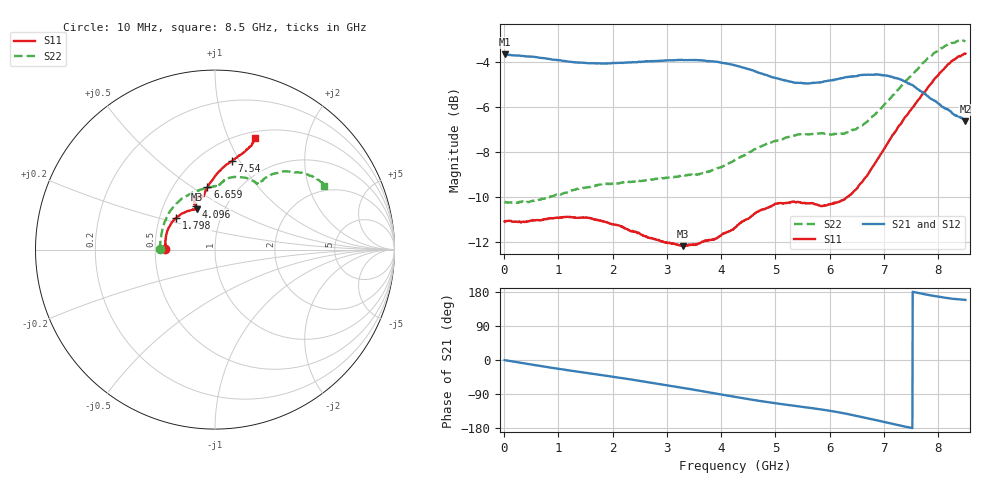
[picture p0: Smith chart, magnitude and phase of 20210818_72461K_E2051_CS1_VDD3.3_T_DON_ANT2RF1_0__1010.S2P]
!Agilent Technologies,E5071C,MY46417908,A.11.23
!Date: Wed Aug 18 14:23:28 2021
!Data & Calibration Information:
!Freq	S11:SOLT2(ON)	S21:SOLT2(ON)	S12:SOLT2(ON)	S22:SOLT2(ON)
!PortZ  Port1:50+j0  Port2:50+j0
!Above PortZ is port z conversion or system Z0 setting when saving the data.
!When reading, reference impedance value at option line is always used.
# Hz S dB R 50
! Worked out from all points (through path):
!   1601 points, 10 MHz to 8.5 GHz, reference 50 ohm
!   highest |S21| = -3.64 dB at 10 MHz (marker M1); lowest = -6.6 dB at 8.5 GHz (marker M2)
!   group delay of S21, straight-line fit = 65.9 ps
!   lowest |S11| = -12.2 dB at 3.3 GHz (marker M3), VSWR 1.65, Z = 37.3 + j17.8 ohm
!   |S11| at or under -10 dB: start of sweep to 6.323 GHz
!   |S22| runs from -10.3 to -3.0 dB; largest |S21 - S12| = 0.0034
!   S11 on the Smith chart (normalised r, x): 10 MHz: 0.56, +0.00; 1.798 GHz: 0.61, +0.23; 4.096 GHz: 0.72, +0.37; 6.659 GHz: 0.73, +0.58; 7.54 GHz: 0.70, +0.93; 8.5 GHz: 0.57, +1.26
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1e7  -11.09 179.7  -3.64 -0.4  -3.64 -0.4  -10.21 179.8
5.671562e8  -11.05 169.9  -3.76 -13.4  -3.76 -13.4  -10.17 163.7
9.704312e8  -10.92 161.6  -3.89 -22.6  -3.88 -22.6  -9.89 151.5
1.426769e9  -10.92 150.6  -4.01 -32.2  -4.01 -32.2  -9.61 136.6
1.798206e9  -11.07 141.0  -4.04 -39.9  -4.05 -39.9  -9.43 124.3
2.238625e9  -11.41 130.3  -4.01 -49.2  -4.01 -49.2  -9.33 111.1
2.843538e9  -11.93 118.3  -3.93 -62.8  -3.93 -62.9  -9.18 96.7
3.299875e9  -12.19 113.8  -3.90 -73.7  -3.89 -73.7  -9.05 90.1
3.6607e9  -11.99 113.0  -3.91 -82.6  -3.91 -82.6  -8.94 87.0
4.095812e9  -11.58 114.3  -4.04 -93.4  -4.04 -93.4  -8.56 84.6
4.255e9  -11.37 114.0  -4.13 -97.3  -4.12 -97.3  -8.35 83.1
4.615825e9  -10.75 113.6  -4.39 -105.9  -4.39 -105.8  -7.88 79.7
5.008488e9  -10.31 110.9  -4.70 -114.2  -4.71 -114.2  -7.50 73.7
5.671769e9  -10.28 104.3  -4.92 -127.0  -4.94 -127.0  -7.20 62.4
6.228925e9  -10.16 101.4  -4.70 -139.7  -4.71 -139.8  -7.18 57.3
6.658731e9  -9.12 96.9  -4.55 -152.5  -4.54 -152.6  -6.70 55.7
7.088538e9  -7.51 88.7  -4.61 -166.4  -4.61 -166.4  -5.67 53.1
7.316706e9  -6.72 84.0  -4.77 -173.6  -4.77 -173.6  -5.05 50.3
7.539569e9  -5.97 79.1  -5.04 179.6  -5.03 179.6  -4.51 47.0
8.022438e9  -4.48 71.7  -5.86 166.3  -5.83 166.4  -3.41 37.4
8.346119e9  -3.78 70.2  -6.39 160.5  -6.36 160.6  -3.05 32.1
8.5e9  -3.61 70.1  -6.63 158.6  -6.57 158.6  -3.07 30.4
